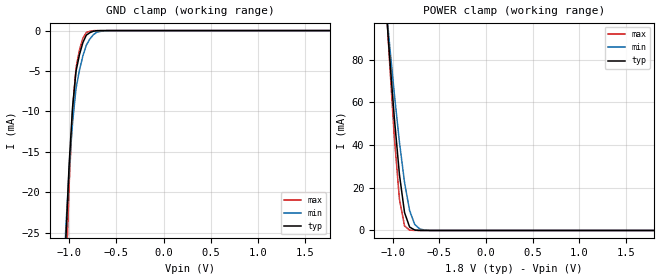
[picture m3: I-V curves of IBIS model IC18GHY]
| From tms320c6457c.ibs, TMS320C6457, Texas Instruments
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|   Model Cell IC18GHY
|IC18GHY_1P8
[Model]   IC18GHY
Model_type   Input
Polarity   Non-Inverting
| Cell operated at 1.8(nom)
| BUFFER OPERATING IN NORMAL MODE WITH +/- 5% VDDS
Vinl =  0.63
Vinh =  1.17
C_comp   0.6553126p   0.5625202p   0.7723385p
[Model Spec]
Vinl   0.63   0.5985   0.6615
Vinh   1.17   1.1115   1.2285
[Temperature Range]   25   125   -40
[Voltage Range]   1.8   1.71   1.89
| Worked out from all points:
|   GND clamp passes 1 mA (typ) near -0.84 V on its own axis
|   POWER clamp passes 1 mA (typ) near -0.79 V on its own axis
[POWER_clamp]
|   voltage   I(typ)   I(min)   I(max)
-1.8V     607mA      492.8mA    733.5mA
-1.055V   94.75mA    97.21mA    95.13mA
-1.036V   83.56mA    88.51mA    81.22mA
-981.8mV  52.51mA    63.81mA    43.47mA
-927.3mV  26.09mA    41.33mA    14.63mA
-872.7mV  8.397mA    22.47mA    2.133mA
-818.2mV  1.587mA    9.312mA    180.8uA
-763.6mV  228.2uA    2.824mA    13.3uA
-709.1mV  29.94uA    699uA      954.2nA
-654.5mV  3.826uA    158.9uA    68.5nA
1.8V      3.537pA    1.47pA     16.1pA
[GND_clamp]
|   voltage   I(typ)   I(min)   I(max)
-1.8V     -539.1mA   -380.2mA   -748.9mA
-1.036V   -26.23mA   -24.68mA   -32.15mA
-1V       -16.52mA   -17.21mA   -19.02mA
-963.6mV  -9.451mA   -11.37mA   -9.842mA
-927.3mV  -5.032mA   -7.151mA   -4.619mA
-890.9mV  -2.977mA   -4.906mA   -2.412mA
-854.5mV  -1.487mA   -3.125mA   -949uA
-818.2mV  -563.1uA   -1.808mA   -231uA
-781.8mV  -269.9uA   -1.064mA   -91.3uA
-709.1mV  -19.12uA   -213.6uA   -1.453uA
-600mV    -278.7nA   -13.18uA   -6.862nA
1.764V    3.096pA    9.108pA    10.16pA
